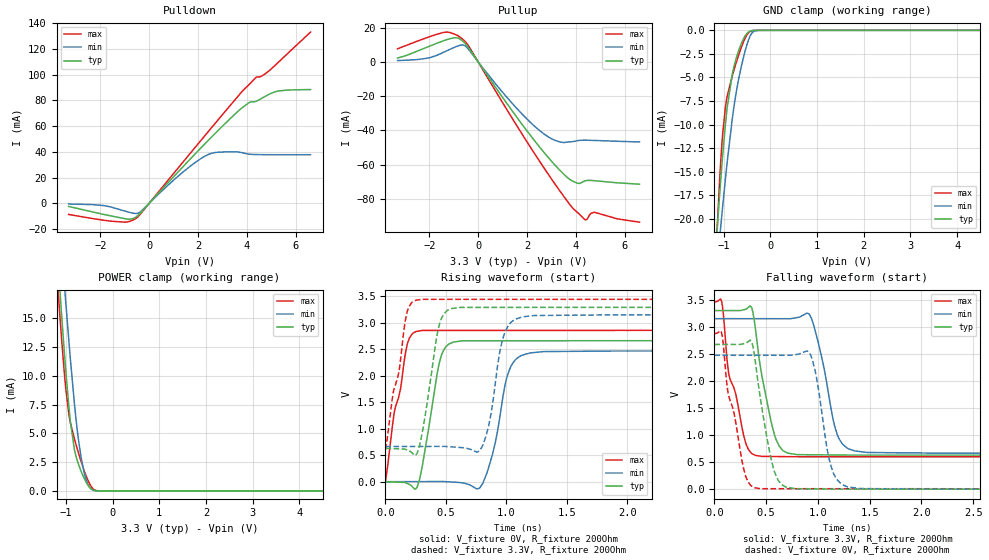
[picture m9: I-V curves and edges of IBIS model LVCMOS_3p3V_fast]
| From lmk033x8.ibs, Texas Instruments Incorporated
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[Model]   LVCMOS_3p3V_fast
Model_type   3-state
Polarity   Non-Inverting
Vmeas = 1.65
Vref = 3.3
Cref = 15pF
Rref = 200
|   typ   min   max
|   (nom PVT)   (fast PVT)   (slow PVT)
C_comp   0.573p   0.551p   0.631p
|C_comp (ON state)   0.666p   0.628p   0.716p
|C_comp (OFF state)   0.573p   0.551p   0.631p
[Voltage Range]   3.3   3.15   3.45
[Temperature Range]   27   125   -40
[Pullup Reference]   3.3   3.15   3.45
[Pulldown Reference]   0   0   0
[Power Clamp Reference]   3.3   3.15   3.45
[GND Clamp Reference]   0   0   0
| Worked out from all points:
|   slope of the pulldown table from 0 to 0.495 V, typ, clamps not added: 48 ohm
|   slope of the pullup table from 0 to 0.495 V, typ, clamps not added: 47.7 ohm
|   GND clamp passes 1 mA (typ) near -0.58 V on its own axis
|   POWER clamp passes 1 mA (typ) near -0.60 V on its own axis
|   falling waveform, V_fixture 3.3V, R_fixture 200Ohm: 20-80 % time 149ps typ, 152ps min, 162ps max; typ from 3.3 V to 0.629 V
|   rising waveform, V_fixture 0V, R_fixture 200Ohm: 20-80 % time 113ps typ, 123ps min, 123ps max; typ from 0.001 V to 2.67 V
|   rising waveform, V_fixture 3.3V, R_fixture 200Ohm: 20-80 % time 104ps typ, 102ps min, 119ps max; typ from 0.63 V to 3.3 V
|   falling waveform, V_fixture 0V, R_fixture 200Ohm: 20-80 % time 140ps typ, 123ps min, 158ps max; typ from 2.67 V to 0 V
[Pulldown]
|   Voltage   I(typ)   I(min)   I(max)
-3.3V     -2.52mA    -600.3uA   -8.758mA
-1.865V   -8.706mA   -1.855mA   -13.25mA
-963.6mV  -12.15mA   -6.33mA    -14.77mA
-528mV    -10.55mA   -7.967mA   -11.61mA
-379.5mV  -7.92mA    -6.939mA   -8.819mA
1.541V    31.66mA    26.77mA    35.73mA
2.511V    50.79mA    38.65mA    57.96mA
3.482V    68.92mA    40.03mA    79.92mA
4.125V    78.74mA    38.11mA    93.15mA
4.372V    79.36mA    37.88mA    97.98mA
5.273V    87.34mA    37.74mA    109.6mA
6.6V      88.5mA     37.75mA    133.2mA
[GND Clamp]
|   Voltage   I(typ)   I(min)   I(max)
-3.3V     -203.8mA   -156.3mA   -307mA
-1.171V   -23.41mA   -26.67mA   -23.99mA
-1.073V   -16.48mA   -21.32mA   -14.64mA
-1.053V   -15.2mA    -20.29mA   -13.1mA
-1.023V   -13.35mA   -18.76mA   -11.08mA
-963.6mV  -10.02mA   -15.81mA   -8.174mA
-924mV    -8.154mA   -13.94mA   -6.971mA
-815.1mV  -4.636mA   -9.357mA   -4.815mA
-636.9mV  -1.582mA   -4.164mA   -2.006mA
-438.9mV  -95.08uA   -660.3uA   -145.6uA
-260.7mV  -658.8nA   -9.216uA   -902.5nA
6.6V      0A         0A         0A
[Pullup]
|   Voltage   I(typ)   I(min)   I(max)
-3.3V     2.259mA    815.6uA    7.66mA
-2.072V   8.734mA    2.189mA    14.32mA
-1.439V   12.24mA    5.483mA    17.14mA
-815.1mV  13.98mA    9.403mA    15.2mA
-468.6mV  9.775mA    8.571mA    10.86mA
1.264V    -26.02mA   -22.09mA   -29.92mA
2.511V    -49.62mA   -40mA      -57.94mA
3.204V    -61.15mA   -46.09mA   -72.5mA
3.897V    -69.75mA   -46.44mA   -85.74mA
4.402V    -69.29mA   -45.69mA   -92.17mA
4.749V    -69.29mA   -45.82mA   -87.72mA
6.6V      -71.34mA   -46.7mA    -93.52mA
[POWER Clamp]
|   Voltage   I(typ)   I(min)   I(max)
-3.3V     163.1mA    154.7mA    175.2mA
-1.162V   19.42mA    25.01mA    17.09mA
-1.092V   15.36mA    21.2mA     13.24mA
-1.013V   11.02mA    16.97mA    9.368mA
-933.9mV  7.229mA    12.94mA    6.584mA
-904.2mV  6.039mA    11.5mA     5.927mA
-815.1mV  3.558mA    7.522mA    4.491mA
-716.1mV  2.165mA    4.038mA    3.108mA
-656.7mV  1.543mA    2.548mA    2.342mA
-567.6mV  770.8uA    1.019mA    1.318mA
-409.2mV  60.75uA    64.51uA    154.9uA
6.6V      0A         0A         0A
[Ramp]
R_load = 200
|   typ   min   max
dV/dt_r   1.60213/1.12495e-10   1.48245/1.22703e-10   1.70939/1.22666e-10
dV/dt_f   1.60254/1.49199e-10   1.49103/1.52008e-10   1.71296/1.61555e-10
[Falling Waveform]
V_fixture = 3.3V
V_fixture_min = 3.15V
V_fixture_max = 3.45V
R_fixture = 200Ohm
C_fixture = 0F
|   Time   V(typ)   V(min)   V(max)
0s        3.3V       3.15V      3.453V
70.44ps   3.3V       3.15V      3.465V
140.9ps   3.3V       3.15V      2.116V
356.9ps   3.366V     3.15V      665mV
457.8ps   2.111V     3.15V      605.8mV
626.1ps   795.6mV    3.149V     602.4mV
916.1ps   635.9mV    3.234V     598.4mV
1.189ns   631.2mV    996.9mV    598.4mV
1.464ns   629.3mV    680.5mV    598.4mV
19ns      629.2mV    665mV      598.3mV
[Rising Waveform]
V_fixture = 0V
V_fixture_min = 0V
V_fixture_max = 0V
R_fixture = 200Ohm
C_fixture = 0F
|   Time   V(typ)   V(min)   V(max)
0s        959.1uV    65.83nV    15.25mV
179.6ps   -33.08mV   1.244mV    2.586V
304.9ps   299.7mV    2.112mV    2.858V
441ps     2.201V     3.055mV    2.858V
499.7ps   2.549V     429.6uV    2.858V
779ps     2.663V     -117.8mV   2.858V
888.6ps   2.663V     551mV      2.858V
1.033ns   2.663V     2.157V     2.858V
1.3ns     2.663V     2.456V     2.858V
19ns      2.671V     2.471V     2.864V
[Rising Waveform]
V_fixture = 3.3V
V_fixture_min = 3.15V
V_fixture_max = 3.45V
R_fixture = 200Ohm
C_fixture = 0F
|   Time   V(typ)   V(min)   V(max)
0s        630.2mV    665mV      605.6mV
176.6ps   600.3mV    665.5mV    3.181V
249.7ps   499.4mV    665.8mV    3.427V
299.5ps   869.7mV    665.9mV    3.445V
450.7ps   3.01V      666.4mV    3.445V
618.6ps   3.292V     646.2mV    3.445V
803.4ps   3.292V     679.7mV    3.445V
990.1ps   3.293V     2.833V     3.445V
1.226ns   3.293V     3.138V     3.445V
19ns      3.3V       3.15V      3.45V
[Falling Waveform]
|Gnd
V_fixture = 0V
V_fixture_min = 0V
V_fixture_max = 0V
R_fixture = 200Ohm
C_fixture = 0F
|   Time   V(typ)   V(min)   V(max)
0s        2.674V     2.474V     2.869V
72.31ps   2.674V     2.474V     2.868V
133.6ps   2.674V     2.474V     1.769V
356.9ps   2.735V     2.474V     59.99mV
443.4ps   1.691V     2.474V     8.654mV
604.5ps   207.8mV    2.473V     8.579mV
912.4ps   5.837mV    2.535V     8.435mV
1.139ns   1.237mV    346.8mV    8.329mV
1.395ns   102.1uV    13.42mV    8.21mV
19ns      223.2nV    49.31nV    51.45nV
